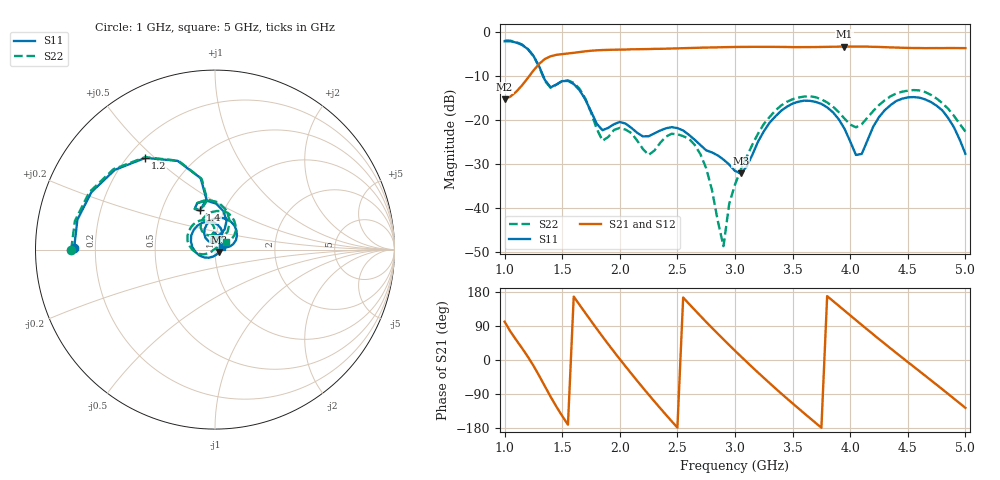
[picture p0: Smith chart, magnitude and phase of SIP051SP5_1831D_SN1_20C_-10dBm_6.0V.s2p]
# GHz  S  dB  R  50
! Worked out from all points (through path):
!   81 points, 1 GHz to 5 GHz, reference 50 ohm
!   highest |S21| = -3.31 dB at 3.95 GHz (marker M1); lowest = -15.3 dB at 1 GHz (marker M2)
!   lowest |S11| = -32.1 dB at 3.05 GHz (marker M3), VSWR 1.05, Z = 52.1 - j1.39 ohm
!   |S11| at or under -10 dB: 1.335 GHz to end of sweep
!   |S22| runs from -48.7 to -1.9 dB; largest |S21 - S12| = 0.0022
!   S11 on the Smith chart (normalised r, x): 1 GHz: 0.12, +0.00; 1.2 GHz: 0.27, +0.47; 1.4 GHz: 0.77, +0.36; 5 GHz: 1.08, +0.03
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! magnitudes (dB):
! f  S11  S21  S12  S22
! 1 GHz  -2.1  -15.3  -15.3  -1.9
! 1.2 GHz  -3.9  -10.5  -10.5  -3.8
! 1.4 GHz  -12.6  -5.5  -5.5  -12.7
! 1.55 GHz  -11.1  -4.9  -4.9  -11.0
! 1.7 GHz  -15.3  -4.4  -4.4  -15.1
! 1.85 GHz  -22.3  -4.1  -4.1  -24.7
! 2 GHz  -20.4  -4.0  -4.0  -21.8
! 2.25 GHz  -23.7  -3.9  -3.9  -28.0
! 2.35 GHz  -22.4  -3.8  -3.8  -25.2
! 2.65 GHz  -24.5  -3.6  -3.6  -25.6
! 2.75 GHz  -26.9  -3.5  -3.5  -31.0
! 2.9 GHz  -29.0  -3.5  -3.5  -48.7
! 2.95 GHz  -30.1  -3.4  -3.4  -39.0
! 3 GHz  -31.6  -3.4  -3.4  -34.7
! 3.05 GHz  -32.1  -3.4  -3.4  -31.3
! 3.35 GHz  -19.2  -3.4  -3.4  -17.9
! 3.7 GHz  -15.9  -3.4  -3.4  -14.8
! 3.95 GHz  -21.9  -3.3  -3.3  -19.7
! 4.1 GHz  -27.7  -3.3  -3.3  -21.0
! 4.35 GHz  -16.6  -3.5  -3.5  -14.6
! 4.75 GHz  -16.8  -3.7  -3.7  -15.1
! 5 GHz  -27.7  -3.7  -3.7  -22.6
